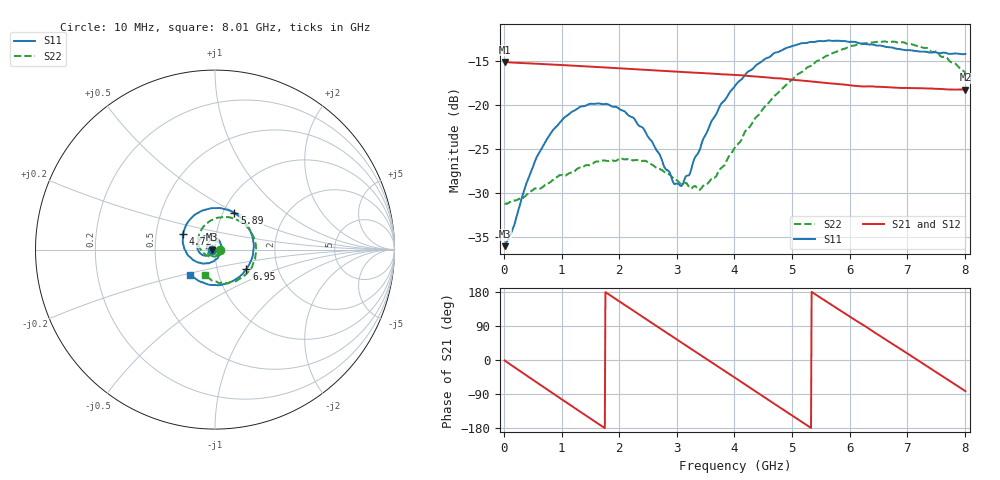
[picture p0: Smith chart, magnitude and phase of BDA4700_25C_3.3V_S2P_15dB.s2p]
!Agilent Technologies,E5071B,MY42404982,A.09.10
!Date: Mon Oct 20 18:09:20 2025
!Data & Calibration Information:
!Freq	S11:SOLT2(ON)	S21:SOLT2(ON)	S12:SOLT2(ON)	S22:SOLT2(ON)
# Hz S RI R 50
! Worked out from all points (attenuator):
!   801 points, 10 MHz to 8.01 GHz, reference 50 ohm
!   highest |S21| = -15.10 dB at 10 MHz (marker M1); lowest = -18.3 dB at 8.01 GHz (marker M2)
!   lowest |S11| = -36.1 dB at 10 MHz (marker M3), VSWR 1.03, Z = 48.5 - j0.117 ohm
!   |S11| at or under -10 dB: start of sweep to end of sweep
!   |S22| runs from -31.3 to -12.8 dB; largest |S21 - S12| = 0.0021
!   S11 on the Smith chart (normalised r, x): 10 MHz: 0.97, -0.00; 4.72 GHz: 0.69, +0.12; 5.89 GHz: 1.13, +0.49; 6.95 GHz: 1.39, -0.31; 8.01 GHz: 0.73, -0.21
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1e7  -0.0156 -0.0012  0.1758 -0.00386  0.1758 -0.00395  0.0274 -0.00102
1.5e8  -0.0169 -0.00999  0.1676 -0.0479  0.1676 -0.0479  0.0272 -0.00786
6e8  -0.0407 -0.0335  0.0794 -0.1521  0.0793 -0.1521  0.0115 -0.0313
1.01e9  -0.0789 -0.024  -0.0422 -0.1634  -0.0422 -0.1635  -0.0199 -0.0346
1.35e9  -0.0979 0.00812  -0.1261 -0.1087  -0.1261 -0.1088  -0.0418 -0.0139
1.72e9  -0.0862 0.0527  -0.1635 -0.00887  -0.1637 -0.00892  -0.0447 0.0184
2.08e9  -0.048 0.0789  -0.1346 0.0886  -0.1347 0.0884  -0.0233 0.0431
2.42e9  -0.00171 0.0735  -0.0605 0.1466  -0.0605 0.1466  0.00786 0.0474
2.68e9  0.0256 0.047  0.01 0.1566  0.00984 0.1566  0.0267 0.0339
2.95e9  0.0349 0.00724  0.0792 0.1334  0.0789 0.133  0.0358 0.0126
3.08e9  0.0322 -0.0125  0.107 0.1111  0.1059 0.1118  0.0354 -0.000107
3.41e9  0.000768 -0.0571  0.1482 0.0351  0.1482 0.0351  0.0189 -0.0271
3.75e9  -0.0603 -0.0782  0.1402 -0.0529  0.1403 -0.0529  -0.0155 -0.0402
4.01e9  -0.1115 -0.0634  0.1014 -0.1084  0.1016 -0.1081  -0.0475 -0.0321
4.72e9  -0.179 0.0872  -0.0673 -0.125  -0.0668 -0.1255  -0.0923 0.0678
5.35e9  -0.0609 0.2205  -0.136 0.00304  -0.1359 0.00224  -0.0061 0.1681
5.89e9  0.1078 0.2046  -0.0758 0.1067  -0.0759 0.1062  0.131 0.162
6.28e9  0.1936 0.1105  0.00409 0.1275  0.00589 0.1269  0.2084 0.0831
6.68e9  0.2118 -0.0239  0.0832 0.0945  0.0836 0.0944  0.226 -0.0295
6.95e9  0.1754 -0.1072  0.1155 0.048  0.1157 0.0472  0.2019 -0.1034
7.47e9  0.0271 -0.198  0.1085 -0.0596  0.1085 -0.0597  0.0763 -0.186
8.01e9  -0.1365 -0.1394  0.0164 -0.1212  0.0169 -0.1212  -0.0572 -0.1414
